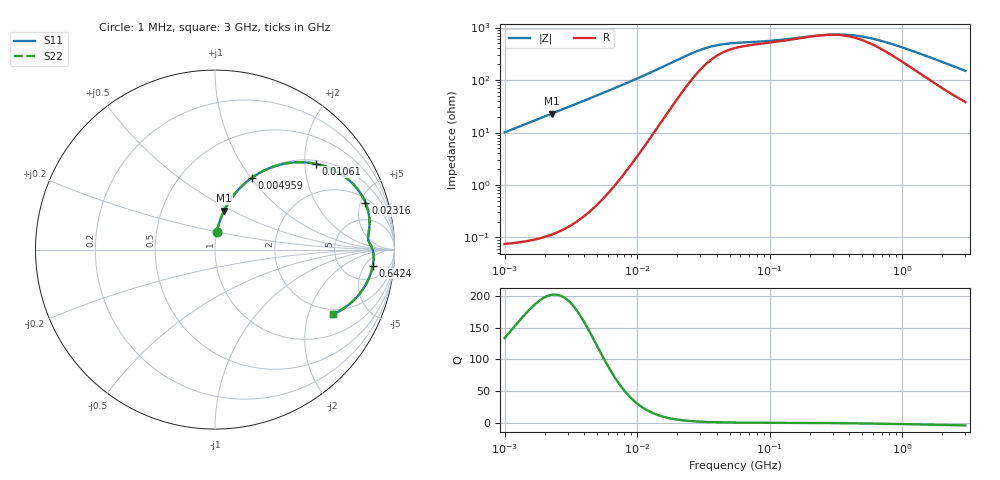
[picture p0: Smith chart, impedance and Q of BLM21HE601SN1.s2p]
! BLM21HE601SN1
# Hz S RI R 50
!Freq.(Hz) S11(Real) S11(Imag) S21(Real) S21(Imag) S12(Real) S12(Imag) S22(Real) S22(Imag)
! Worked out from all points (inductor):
!   401 points, 1 MHz to 3 GHz, reference 50 ohm
!   read as one part in series: L = 1.6 uH near 1.041 MHz
!   highest Q = 202 at 2.272 MHz (marker M1), where L = 1.61 uH
!   self-resonance near 254.9 MHz
!   S11 on the Smith chart (normalised r, x): 1 MHz: 1.00, +0.20; 4.959 MHz: 1.01, +1.01; 10.61 MHz: 1.09, +2.29; 23.16 MHz: 2.43, +5.54; 642.4 MHz: 10, -8; 3 GHz: 1.76, -2.89
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1000000  0.0108 0.0995  0.9892 -0.0995  0.9892 -0.0995  0.0108 0.0995
2271982  0.0509 0.2174  0.9491 -0.2174  0.9491 -0.2174  0.0509 0.2174
3823119  0.1326 0.3361  0.8674 -0.3361  0.8674 -0.3361  0.1326 0.3361
4959344  0.2065 0.4007  0.7935 -0.4007  0.7935 -0.4007  0.2065 0.4007
7550455  0.385 0.478  0.615 -0.478  0.615 -0.478  0.385 0.478
1.061086e7  0.5642 0.4774  0.4358 -0.4774  0.4358 -0.4774  0.5642 0.4774
1.461624e7  0.7163 0.4112  0.2837 -0.4112  0.2837 -0.4112  0.7163 0.4112
1.821614e7  0.7905 0.3411  0.2095 -0.3411  0.2095 -0.3411  0.7905 0.3411
2.316168e7  0.8382 0.2609  0.1618 -0.2609  0.1618 -0.2609  0.8382 0.2609
3.597591e7  0.8611 0.1461  0.1389 -0.1461  0.1389 -0.1461  0.8611 0.1461
4.394807e7  0.859 0.1127  0.141 -0.1127  0.141 -0.1127  0.859 0.1127
5.477226e7  0.8553 0.0872  0.1447 -0.0872  0.1447 -0.0872  0.8553 0.0872
1.103592e8  0.8567 0.0456  0.1433 -0.0456  0.1433 -0.0456  0.8567 0.0456
2.094008e8  0.8734 0.0133  0.1266 -0.0133  0.1266 -0.0133  0.8734 0.0133
2.884452e8  0.8804 -0.00931  0.1196 0.00931  0.1196 0.00931  0.8804 -0.00931
3.741707e8  0.8835 -0.0313  0.1165 0.0313  0.1165 0.0313  0.8835 -0.0313
4.853736e8  0.8835 -0.057  0.1165 0.057  0.1165 0.057  0.8835 -0.057
6.423554e8  0.8793 -0.0895  0.1207 0.0895  0.1207 0.0895  0.8793 -0.0895
8.005644e8  0.8721 -0.1192  0.1279 0.1192  0.1279 0.1192  0.8721 -0.1192
1.645649e9  0.8049 -0.2471  0.1951 0.2471  0.1951 0.2471  0.8049 -0.2471
2.177892e9  0.7482 -0.3044  0.2518 0.3044  0.2518 0.3044  0.7482 -0.3044
3e9  0.6549 -0.3614  0.3451 0.3614  0.3451 0.3614  0.6549 -0.3614
